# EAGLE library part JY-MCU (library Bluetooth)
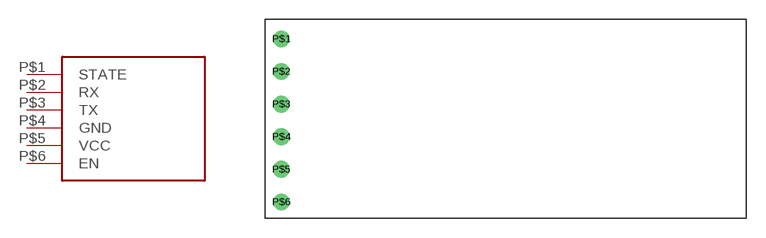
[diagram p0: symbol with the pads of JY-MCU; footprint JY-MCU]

Designator prefix -

## JY-MCU  [JY-MCU]
P$1  STATE  out
P$2  RX  in
P$3  TX  out
P$4  GND  pwr
P$5  VCC  pwr
P$6  EN  in

## Footprint JY-MCU (pad centres in mm)
drill 0.8: P$1 1.27,13.97; P$2 1.27,11.43; P$3 1.27,8.89; P$4 1.27,6.35; P$5 1.27,3.81; P$6 1.27,1.27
